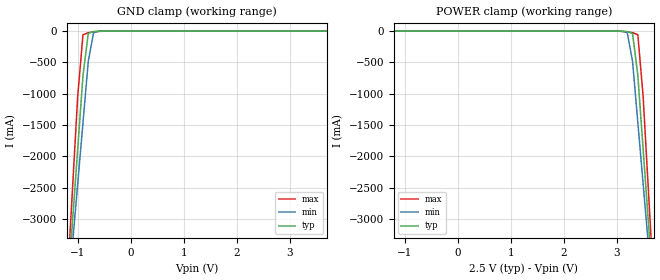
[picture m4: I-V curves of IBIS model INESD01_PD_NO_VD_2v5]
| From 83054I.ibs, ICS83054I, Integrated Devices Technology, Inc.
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[Model] INESD01_PD_NO_VD_2v5
Model_type   Input
Polarity   Non-Inverting
Vinl = 0.80V
Vinh = 2.0V
|   typ   min   max
C_comp   2pF   1.5pF   2.5pF
|   typ   min   max
[Voltage range]  2.5V   2.375V   2.625V
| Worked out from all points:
|   GND clamp passes 1 mA (typ) near -0.53 V on its own axis
[GND_clamp]
|Voltage I(typ)   I(min)   I(max)
-2.5V     -19.61A    -17.19A    -23.68A
-1.2V     -4.247A    -4.404A    -4.063A
-1.1V     -3.067A    -3.422A    -2.554A
-1V       -1.887A    -2.441A    -1.045A
-900mV    -707.9mA   -1.461A    -58.38mA
-800mV    -36.14mA   -481.4mA   -25.07mA
-700mV    -7.313mA   -24.33mA   -13.7mA
-600mV    -2.207mA   -1.763mA   -5.095mA
-500mV    -388.3uA   -196.9uA   -934.5uA
5V        97.41uA    121.8uA    92.26uA
[POWER_clamp]
|Voltage   I(typ)   I(min)   I(max)
-2.5V     97.41uA    121.8uA    92.26uA
3V        -388.3uA   -196.9uA   -934.5uA
3.1V      -2.207mA   -1.763mA   -5.095mA
3.2V      -7.314mA   -24.33mA   -13.7mA
3.3V      -36.14mA   -481.4mA   -25.07mA
3.4V      -707.9mA   -1.461A    -58.38mA
3.5V      -1.887A    -2.441A    -1.045A
3.6V      -3.067A    -3.422A    -2.554A
3.7V      -4.247A    -4.404A    -4.063A
5V        -19.61A    -17.19A    -23.68A
